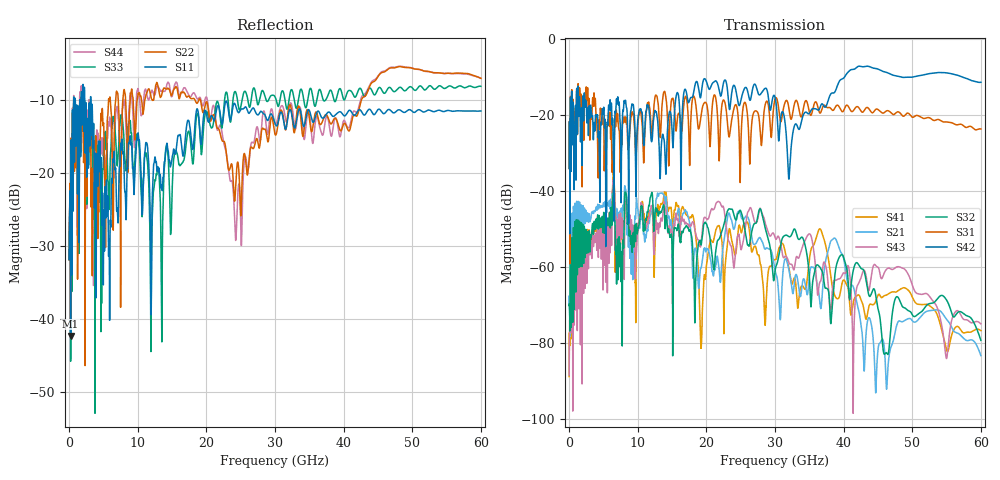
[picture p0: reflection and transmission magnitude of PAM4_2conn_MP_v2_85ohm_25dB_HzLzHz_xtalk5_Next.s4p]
! Info: Touchstone file created by Circ.  Input file=FAB50GbE_2conn_Midplane_Examax_Topo2_v2_85ohm_25dB_HzLzHz.circ
# Hz S RI R 50
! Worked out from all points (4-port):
!   6000 points, 10 MHz to 60 GHz, reference 50 ohm
!   strongest paths, dB at 10 MHz, 15.01 GHz, 30.01 GHz, 45.01 GHz, 60 GHz:
!     S42: -34.0, -24.0, -15.3, -7.9, -11.4
!     S31: -34.1, -15.7, -15.8, -18.5, -23.7
!     S32: -70.1, -54.9, -61.1, -71.0, -79.3
!     S43: -88.5, -53.7, -52.2, -60.1, -75.0
!     S21: -69.7, -51.4, -60.9, -81.7, -83.3
!     S41: -88.9, -47.5, -58.1, -67.4, -76.7
!   lowest |S11| = -42.3 dB at 230 MHz (marker M1), VSWR 1.02, Z = 50.8 + j0.0463 ohm
!   |S11| at or under -10 dB: start of sweep to 671.9 MHz; 2.284 GHz to 3.122 GHz (838.4 MHz wide, 31 % of centre); 3.173 GHz to end of sweep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
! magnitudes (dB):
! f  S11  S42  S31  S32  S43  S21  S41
! 10 MHz  -31.9  -34.0  -34.1  -70.1  -88.5  -69.7  -88.9
! 230 MHz  -42.3  -15.9  -15.5  -56.4  -62.7  -50.0  -57.0
! 13.97 GHz  -18.2  -29.9  -13.9  -49.2  -44.2  -43.4  -40.7
! 19.26 GHz  -16.1  -14.3  -19.7  -54.1  -53.2  -60.1  -80.8
! 21.74 GHz  -10.8  -12.4  -24.5  -52.8  -42.7  -58.8  -49.1
! 32.06 GHz  -11.6  -36.5  -18.6  -52.0  -59.0  -61.0  -60.5
! 60 GHz  -11.5  -11.4  -23.7  -79.3  -75.0  -83.3  -76.7
